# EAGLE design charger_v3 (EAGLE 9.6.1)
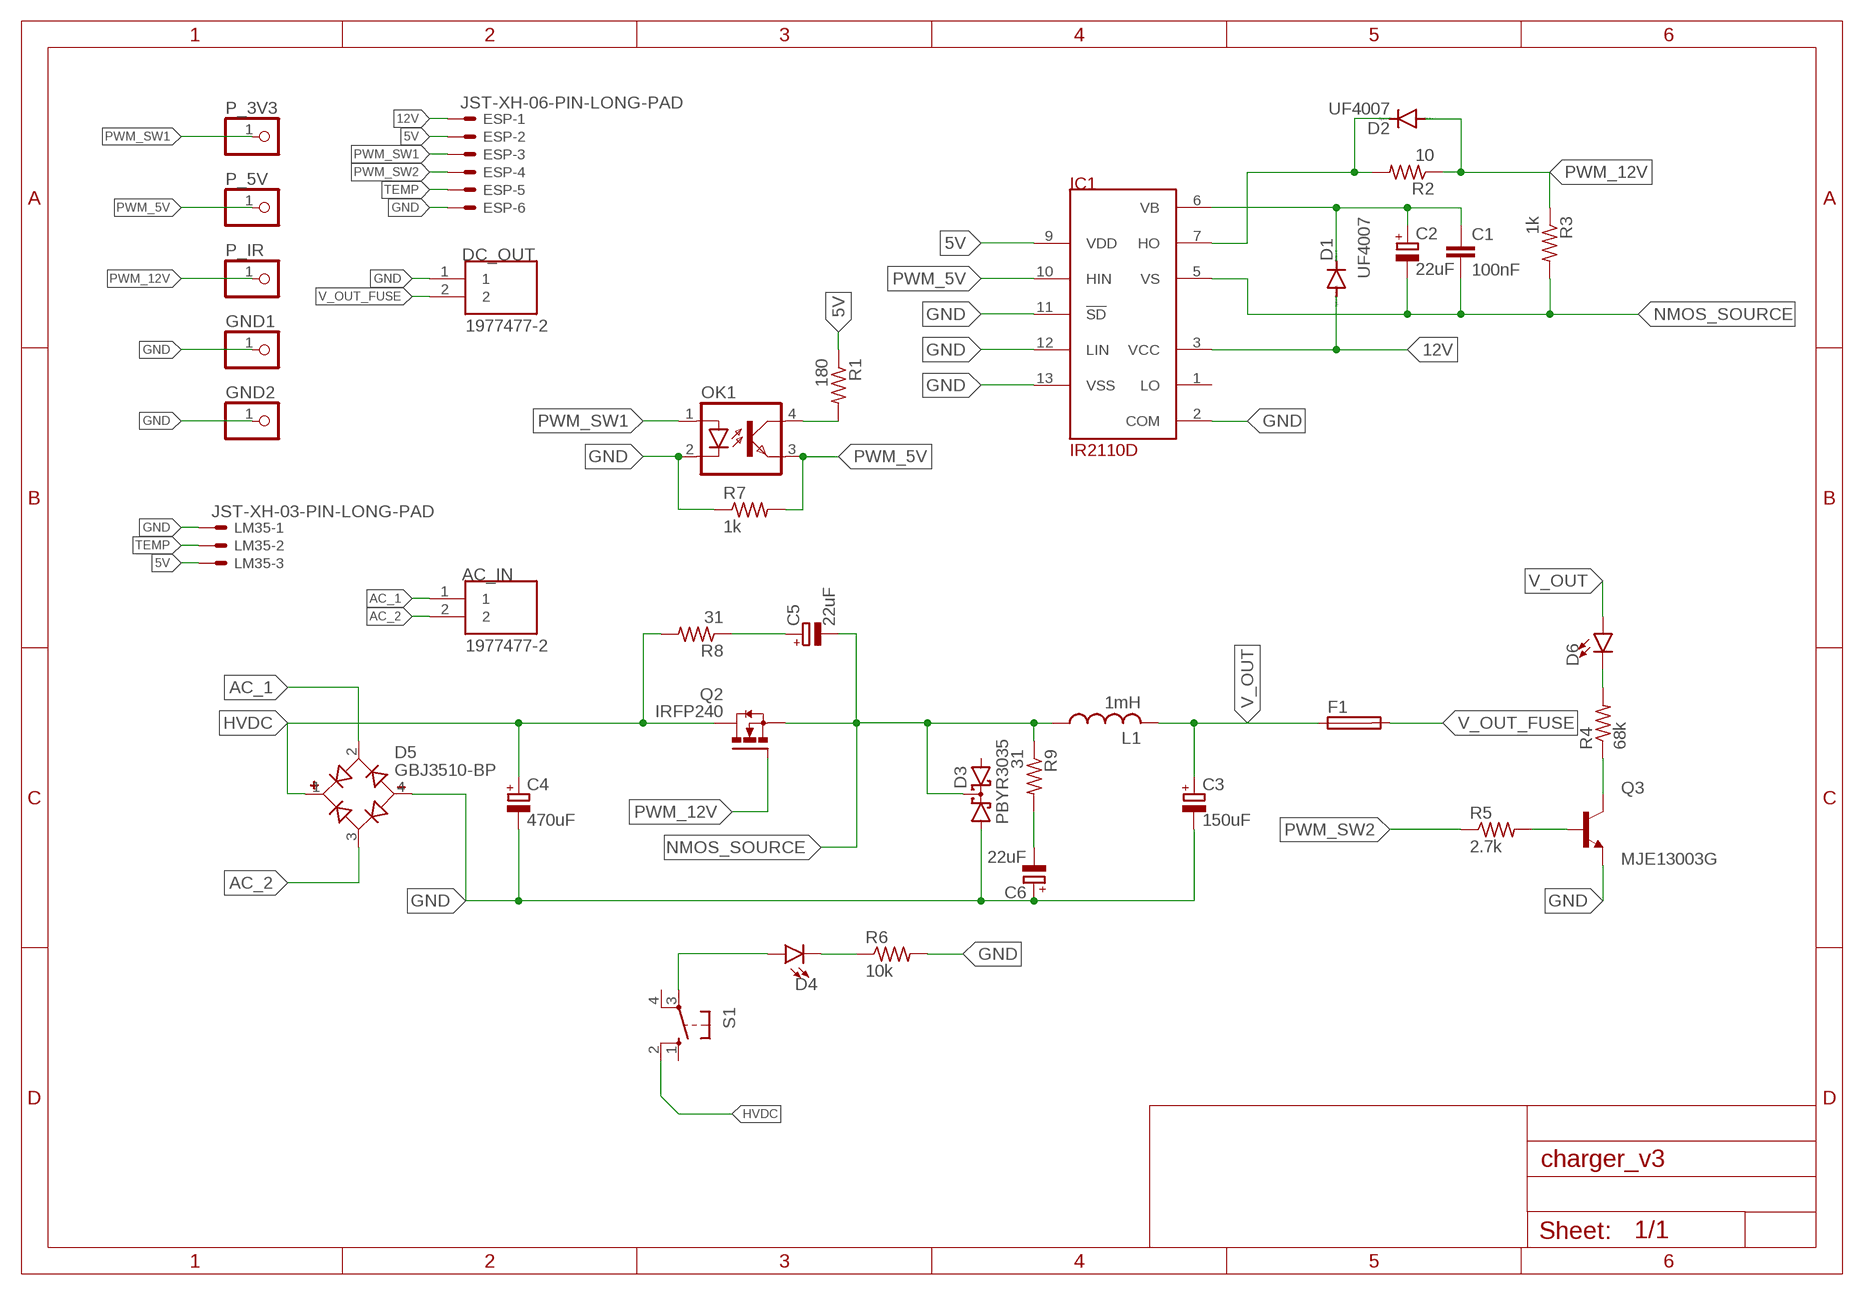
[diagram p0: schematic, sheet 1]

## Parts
AC_IN  1977477-2  [TE_1977477-2]
C1  100nF  C-EU025-025X050  [C025-025X050]
C2  22uF  CPOL-EUE2,5-6E  [E2,5-6E]
C3  150uF  CPOL-EUE7.5-18  [E7,5-18]
C4  470uF  CPOL-EUE10-35  [EB35D]
C5  22uF  CPOL-EUE7.5-18  [E7,5-18]
C6  22uF  CPOL-EUE7.5-18  [E7,5-18]
D1  UF4007  BAS15  [DO34-7]
D2  UF4007  BAS15  [DO34-7]
D3  PBYR3035  [SOT93S]
D4  LED5MM  [LED_5MM]
D5  GBJ3510-BP  [DIOB_GBJ3510-BP]
D6  LED5MM  [LED_5MM]
DC_OUT  1977477-2  [TE_1977477-2]
ESP  JST-XH-06-PIN-LONG-PAD  [JST-XH-06-PACKAGE-LONG-PAD]
F1  FUSEHOLDER  [FUSEHOLDER]
GND1  PINHD-1X1  [1X01]
GND2  PINHD-1X1  [1X01]
IC1  IR2110D  [DIL14]
L1  1mH  L-USTJ7-U1  [TJ7-U1]
LM35  JST-XH-03-PIN-LONG-PAD  [JST-XH-03-PACKAGE-LONG-PAD]
OK1  SFH618A-5  [DIP4]
P_3V3  PINHD-1X1  [1X01]
P_5V  PINHD-1X1  [1X01]
P_IR  PINHD-1X1  [1X01]
Q2  IRFP240  [TO247AC]
Q3  MJE13003G  [TO229P780X300X1364-3]
R1  180  R-US_0204/7  [0204/7]
R2  10  R-US_0204/7  [0204/7]
R3  1k  R-US_0204/7  [0204/7]
R4  68k  R-US_0309/12  [0309/12]
R5  2.7k  R-US_0204/7  [0204/7]
R6  10k  R-US_0204/7  [0204/7]
R7  1k  R-US_0204/7  [0204/7]
R8  31  R-US_0411/15  [0411/15]
R9  31  R-US_0411/15  [0411/15]
S1  10-XX  [B3F-10XX]

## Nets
5V: ESP.2 IC1.9(VDD) LM35.3 R1.1
12V: D1.A ESP.1 IC1.3(VCC)
AC_1 [power]: AC_IN.1 D5.2(AC1)
AC_2 [power]: AC_IN.2 D5.3(AC2)
GND: C3.- C4.- C6.+ D3.A1 D5.4(-) DC_OUT.1 ESP.6 GND1.1 GND2.1 IC1.2(COM) IC1.11(!SD) IC1.12(LIN) IC1.13(VSS) LM35.1 OK1.2(C) Q3.3(E) R6.2 R7.1
HVDC: C4.+ D5.1(+) Q2.2(D) R8.2 S1.2(S1)
N$1: D2.C IC1.7(HO) R2.2
N$2: D4.A S1.3(P)
N$3: Q3.2(C) R4.1
N$4: D6.K(C) R4.2
N$5: Q3.1(B) R5.2
N$6: C5.+ R8.1
N$7: C6.- R9.2
N$8: D4.K(C) R6.1
N$11: OK1.4(COL) R1.2
NMOS_SOURCE: C1.2 C2.- C5.- D3.C IC1.5(VS) L1.1 Q2.3(S) R3.2 R9.1
PWM_5V: IC1.10(HIN) OK1.3(EMIT) P_5V.1 R7.2
PWM_12V [pwm_12]: D2.A P_IR.1 Q2.1(G) R2.1 R3.1
PWM_SW1: ESP.3 OK1.1(A) P_3V3.1
PWM_SW2: ESP.4 R5.1
TEMP: ESP.5 LM35.2
V_OUT: C3.+ D6.A F1.1 L1.2
V_OUT_FUSE [power]: DC_OUT.2 F1.2
VB: C1.1 C2.+ D1.C IC1.6(VB)
Unconnected: D3.A2 IC1.1(LO) S1.1(S) S1.4(P1)

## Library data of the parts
AC_IN DC_OUT = terminal_block_TA:1977477-2: Check availability; AVAILABILITY: In Stock; COMMENT: 1977477-2; DESCRIPTION: Conn Barrier Strip 2 POS 8.25mm Solder ST Thru-Hole 15A/Contact Carton; MF: TE Connectivity; MP: 1977477-2; PACKAGE: None; PRICE: None; PURCHASE-URL: https://pricing.snapeda.com/search/part/1977477-2/?ref=eda
C1 = rcl:C-EU: CAPACITOR, European symbol; SPICEPREFIX: C
C2-C6 = rcl:CPOL-EU: POLARIZED CAPACITOR, European symbol; SPICEPREFIX: C
D1 D2 = diode:BAS15: DIODE
D3 = diode:PBYR3035: Dual DIODE common cathode
D4 D6 = Sparkfun_LED:LED: LED (Generic)
D5 = GBJ3510-BP:GBJ3510-BP: Diode Rectifier Bridge Single 1KV 35A 4-Pin(4+Tab) Case GBJ Bulk/Tube Check availability; AVAILABILITY: In Stock; DESCRIPTION: Bridge Rectifier Single Phase Standard 1 kV Through Hole GBJ; MF: Micro Commercial; MP: GBJ3510-BP; PACKAGE: SIP-4 Micro Commercial Co; PRICE: None; PURCHASE-URL: https://pricing.snapeda.com/search/part/GBJ3510-BP/?ref=eda
ESP = Rembrandt Electronics - JST XH Connectors v1-0:JST-XH-06-PIN: JST XH Connector 2 Pin Wire to board connector. Pitch: 2,54 mm, (0.100") Number of pins: 6 Created by Rembrandt Electronics www.rembrandtelectronics.com
F1 = TA_library:FUSEHOLDER: FUSE HOLDER; MPN: 0031.7701.11; OC_FARNELL: unknown; OC_NEWARK: 04F1224
GND1 GND2 P_3V3 P_5V P_IR = pinhead:PINHD-1X1: PIN HEADER
IC1 = irs:IR2110
L1 = custom_inductor:L-US: INDUCTOR, American symbol; SPICEPREFIX: L
LM35 = Rembrandt Electronics - JST XH Connectors v1-0:JST-XH-03-PIN: JST XH Connector 2 Pin Wire to board connector. Pitch: 2,54 mm, (0.100") Number of pins: 3 Created by Rembrandt Electronics www.rembrandtelectronics.com
OK1 = optocoupler:SFH618?*: Optocoupler, Phototransistor Output, Low Input Current Source: Data sheet; MF: VISHAY/TELEFUNKEN; MPN: SFH618A-5; OC_FARNELL: 1469593; OC_NEWARK: 59K0259
Q2 = IRFP240(TO-247):IRFP240: MOSFET N-CH 200V 20A TO-247AC Check availability; AVAILABILITY: In Stock; DESCRIPTION: N-Channel 200 V 20A (Tc) 150W (Tc) Through Hole TO-247AC; MF: Vishay Siliconix; MP: IRFP240; PACKAGE: TO-247 Vishay Siliconix; PRICE: None
Q3 = MJE13003G:MJE13003G: Bipolar (BJT) Transistor NPN 400V 1.5A 10MHz 1.4W Through Hole TO-225AA Check availability; AVAILABILITY: Not in stock; DESCRIPTION: Bipolar (BJT) Transistor NPN 400 V 1.5 A 10MHz 1.4 W Through Hole TO-126; MF: ON Semiconductor; MP: MJE13003G; PACKAGE: TO-126 ON Semiconductor; PRICE: None
R1-R9 = rcl:R-US_: RESISTOR, American symbol; SPICEPREFIX: R
S1 = switch-omron:10-XX: OMRON SWITCH; MPN: B3F-1000; OC_FARNELL: 176432; OC_NEWARK: 36M3542

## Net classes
0 default: width 0.305 mm
1 power: width 6.985 mm, clearance 0.508 mm to class 0
2 pwm_12: width 0.305 mm, clearance 0.508 mm to class 0, clearance 0.508 mm to class 1

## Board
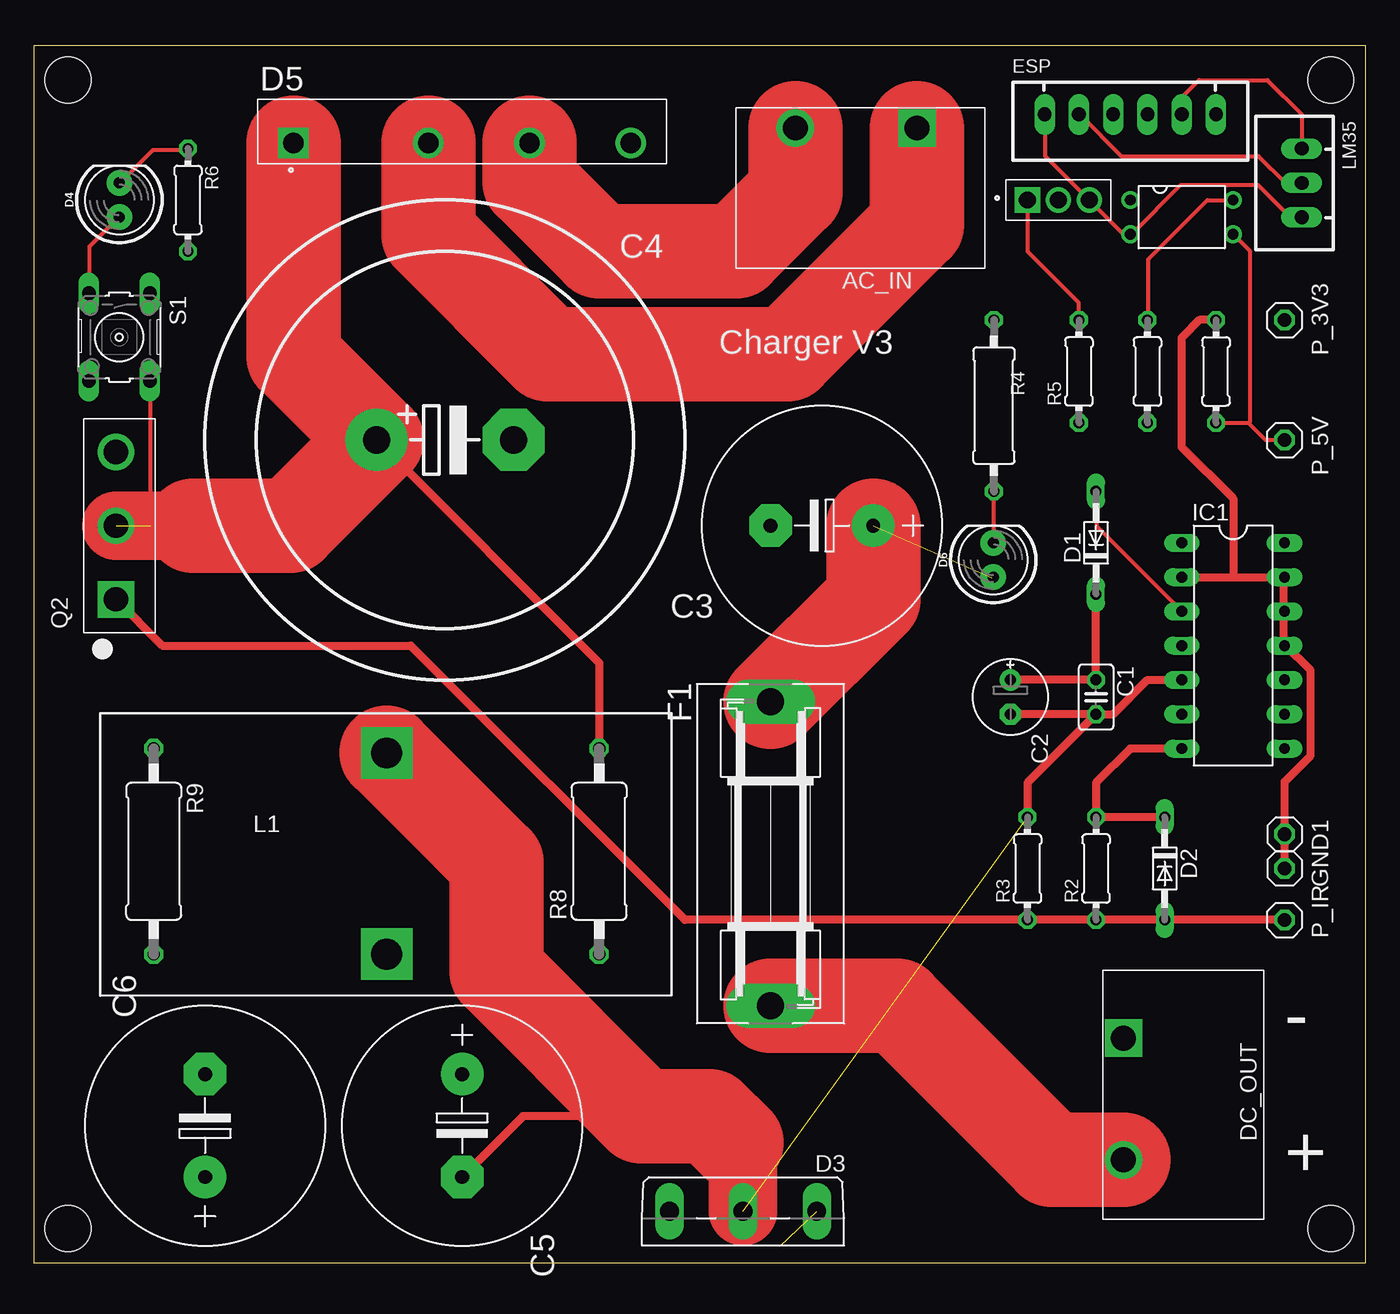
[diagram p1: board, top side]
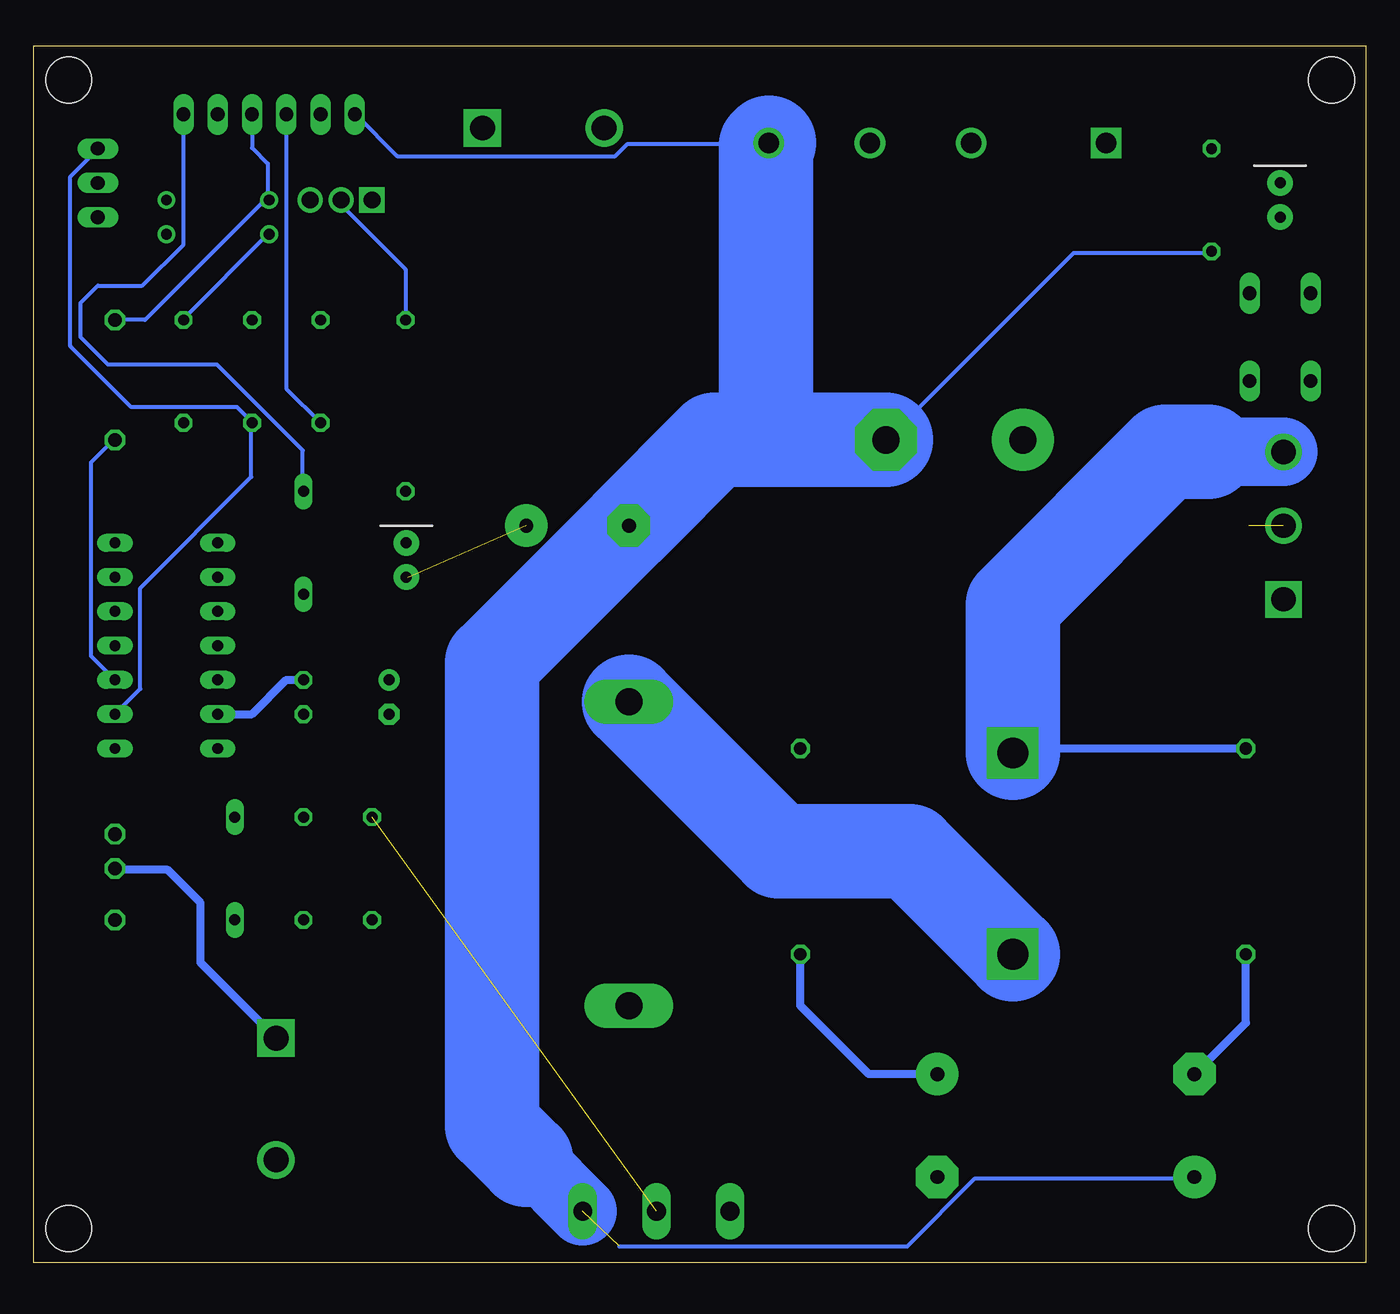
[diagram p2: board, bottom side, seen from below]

Size 98.73 x 90.16 mm. Coordinates in mm from the lower left corner, seen from the top.
Outline: 0,0 98.73,0 98.73,90.16 0,90.16 0,0
Copper layers (1*16): Top 0.035mm / dielectric 1.5mm / Bottom 0.035mm
Design rules "default *": minimum track width 12mil, minimum drill 0.35mm, track to track 12mil, track to pad 12mil, pad to pad 12mil, via to via 12mil, smd to smd 12mil, copper to edge 40mil, drill to drill 6mil, minimum pad ring 10mil, minimum via ring 8mil, stop-mask expansion 4mil, vias tented up to drill 0mil, thermal gap 10mil
Holes 3.4 mm at 2.54,87.63 96.14,87.63 2.54,2.54 96.14,2.54

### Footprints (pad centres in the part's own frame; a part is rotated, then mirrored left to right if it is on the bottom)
TE_1977477-2 = drill 1.85 square: 1 -3.241,-5.334 | drill 1.85: 2 5.781,-5.334
C025-025X050 = drill 0.813 octagon: 1 -1.27,0; 2 1.27,0
E2,5-6E = drill 0.813 pad 1.575: + -1.27,0 | drill 0.813 pad 1.575 octagon: - 1.27,0
E7,5-18 = drill 1.016 pad 3.15: + -3.81,0 | drill 1.016 pad 3.15 octagon: - 3.81,0
EB35D = drill 2.007 pad 4.597: + -5.08,0 | drill 2.007 pad 4.597 octagon: - 5.08,0
DO34-7 = drill 0.813 long: A 3.81,0; C -3.81,0
SOT93S = drill 1.397 long: A1 -5.461,-2.54; A2 5.461,-2.54; C 0,-2.54
LED_5MM = drill 0.813 pad 1.88: A -1.27,0; K 1.27,0
DIOB_GBJ3510-BP = drill 1.51 pad 2.27 square: 1 -12.5,-0.85 | drill 1.51 pad 2.27: 2 -2.5,-0.85; 3 5,-0.85; 4 12.5,-0.85
JST-XH-06-PACKAGE-LONG-PAD = drill 1.016 long: 1 -6.35,0; 2 -3.81,0; 3 -1.27,0; 4 1.27,0; 5 3.81,0; 6 6.35,0
FUSEHOLDER = drill 2.007 pad 3.302 long: 1 -11.252,0; 2 11.252,0
1X01 = drill 1.016 octagon: 1 0,0
DIL14 = drill 0.813 long: 1 -7.62,-3.81; 2 -5.08,-3.81; 3 -2.54,-3.81; 4 0,-3.81; 5 2.54,-3.81; 6 5.08,-3.81; 7 7.62,-3.81; 8 7.62,3.81; 9 5.08,3.81; 10 2.54,3.81; 11 0,3.81; 12 -2.54,3.81; 13 -5.08,3.81; 14 -7.62,3.81
TJ7-U1 = drill 2.286 pad 3.81 square: 1 -6.503,4.826; 2 8.408,4.826
JST-XH-03-PACKAGE-LONG-PAD = drill 1.016 long: 1 -2.54,0; 2 0,0; 3 2.54,0
DIP4 = drill 0.8: 1 -1.27,-3.81; 2 1.27,-3.81; 3 1.27,3.81; 4 -1.27,3.81
TO247AC = drill 1.79 pad 2.69 square: 1 -5.46,0.255 | drill 1.79 pad 2.69: 2 0,0.255; 3 5.46,0.255
TO229P780X300X1364-3 = drill 1.25 square: 1 0,0 | drill 1.25: 2 2.29,0; 3 4.58,0
0204/7 = drill 0.813 octagon: 1 -3.81,0; 2 3.81,0
0309/12 = drill 0.813 octagon: 1 -6.35,0; 2 6.35,0
0411/15 = drill 0.914 octagon: 1 -7.62,0; 2 7.62,0
B3F-10XX = drill 1.016 long: 1 -3.251,2.261; 2 3.251,2.261; 3 -3.251,-2.261; 4 3.251,-2.261

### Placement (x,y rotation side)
AC_IN  62.23,78.74 180 top
C1  78.74,41.91 270 top
C2  72.39,41.91 270 top
C3  58.42,54.61 180 top
C4  30.48,60.96 0 top
C5  31.75,10.16 270 top
C6  12.7,10.16 90 top
D1  78.74,53.34 90 top
D2  83.82,29.21 270 top
D3  52.58,1.27 180 top
D4  6.35,78.74 90 top
D5  31.75,83.82 0 top
D6  71.12,52.07 90 top
DC_OUT  86.11,13.4 270 top
ESP  81.28,85.09 180 top
F1  54.61,30.3 270 top
GND1  92.71,31.75 0 top
GND2  92.71,29.21 0 top
IC1  88.9,45.72 270 top
L1  21.34,31.27 270 top
LM35  93.98,80.01 90 top
OK1  85.09,77.47 270 top
P_3V3  92.71,69.85 90 top
P_5V  92.71,60.96 90 top
P_IR  92.71,25.4 90 top
Q2  6.35,54.61 90 top
Q3  73.66,78.74 0 top
R1  82.55,66.04 90 top
R2  78.74,29.21 90 top
R3  73.66,29.21 90 top
R4  71.17,63.5 270 top
R5  77.47,66.04 90 top
R6  11.43,78.74 270 top
R7  87.63,66.04 270 top
R8  41.91,30.48 90 top
R9  8.89,30.48 270 top
S1  6.35,68.58 270 top

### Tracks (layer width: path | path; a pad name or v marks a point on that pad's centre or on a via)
5V
  Top 0.305: LM35.3 93.98,85.09 91.44,87.63 86.36,87.63 85.09,86.36 ESP.2
  Bottom 0.305: IC1.9 90.83,42.52 90.83,49.99 82.6,58.22 82.6,62.18 R1.1 82.6,62.33 83.67,63.4 91.49,63.4 96.01,67.92 96.01,80.47 94.03,82.45 LM35.3
12V
  Top 0.305: IC1.3 78.79,54.56 78.79,57.15 D1.A
  Bottom 0.305: ESP.1 87.63,75.44 90.68,72.39 93.98,72.39 95.25,71.12 95.25,68.58 93.22,66.55 85.14,66.55 78.79,60.2 78.79,57.15 D1.A
AC_1
  Top 6.985: AC_IN.1 65.47,76.9 55.88,67.31 38.1,67.31 29.25,76.16 D5.2
AC_2
  Top 6.985: AC_IN.2 56.45,79.31 52.07,74.93 41.91,74.93 36.75,80.09 D5.3
GND  (1 unrouted)
  Top 0.305: 54.56,54.71 C3.- | 35.66,60.96 C4.- | GND2.1 92.81,29.26 92.81,31.7 GND1.1 92.81,31.85 92.81,35.81 94.49,37.49 94.49,44.04 92.81,45.72 IC1.11 92.66,45.72 92.66,48.16 IC1.12 92.66,48.31 92.66,50.75 IC1.13 92.66,50.9 | ESP.6 74.98,85.04 74.98,81.99 78.18,78.79 Q3.3 78.33,78.64 80.77,76.2 OK1.2 81.38,76.2 85.04,79.86 90.73,79.86 93.02,77.57 93.88,77.57 LM35.1
  Top 0.61: GND2.1 92.71,35.64 94.64,37.57 94.64,43.89 92.81,45.72 | IC1.11 92.66,45.77 92.66,50.9 92.56,50.8 88.9,50.8 | 88.9,50.8 88.9,56.62 85.09,60.43 85.09,68.53 86.41,69.85 R7.1 | IC1.2 88.9,50.8
  Bottom 0.305: R6.2 11.43,74.83 21.64,74.83 35.51,60.96 C4.- | 44.2,82.91 D5.4 44.35,82.91 54.71,82.91 55.63,81.99 71.78,81.99 74.83,85.04 ESP.6 | R7.1 87.63,69.95 81.38,76.2 OK1.2 | 55.32,1.22 33.98,1.22 28.96,6.25 12.8,6.25 C6.+
  Bottom 0.61: GND2.1 92.61,29.11 88.8,29.11 86.36,26.67 86.36,22.23 DC_OUT.1
  Bottom 3.81: 64.39,10.16 64.77,10.16
  Bottom 5.08: D3.A1 61.85,7.62 62.23,7.62
  Bottom 6.985: 62.23,7.62 64.77,10.16 64.77,44.45 C3.- 48.26,60.96 44.45,60.96 | C4.- 44.45,60.96 | D5.4 44.45,82.77 44.45,60.96
HVDC  (1 unrouted)
  Top 0.305: 8.69,54.61 8.69,65.23 S1.2
  Top 0.61: R8.2 41.91,44.45 C4.+
  Top 5.08: Q2.2 11.81,54.61
  Top 6.985: D5.1 19.25,67.11 C4.+ 19.05,54.61 11.81,54.61
N$1
  Top 0.61: IC1.7 81.28,38.1 78.74,35.56 R2.2 D2.C
N$2
  Top 0.305: S1.3 4.12,71.93 4.12,75.29 6.25,77.42 D4.A
N$3
  Bottom 0.305: R4.1 71.17,73.61 75.89,78.33 75.89,78.64 Q3.2
N$4
  Top 0.305: R4.2 71.17,53.34 D6.K
N$5
  Top 0.305: Q3.1 73.66,74.93 77.42,71.17 77.42,69.95 R5.2
N$6
  Bottom 0.61: C5.+ 36.83,13.97 41.91,19.05 R8.1
N$7
  Bottom 0.61: C6.- 8.89,17.78 R9.2
N$8
  Top 0.305: R6.1 11.43,82.45 8.84,82.45 6.4,80.01 D4.K
N$11
  Top 0.305: OK1.4 87,78.74 82.6,74.35 82.6,72.75 82.6,72.39 82.6,69.95 R1.2
NMOS_SOURCE  (1 unrouted)
  Top 0.61: C1.2 80.01,40.64 82.55,43.18 IC1.5 | C1.2 C2.- | C1.2 73.66,35.56 R3.2 | 45.02,10.86 36.26,10.86 C5.-
  Top 5.08: D3.C 52.58,8.38 52.07,8.89
  Top 6.985: L1.1 34.29,29.64 34.29,21.59 45.02,10.86 50.1,10.86 52.07,8.89
  Bottom 0.61: R9.1 25.83,38.1 L1.1
  Bottom 5.08: Q2.3 11.68,60.07
  Bottom 6.985: L1.1 26.16,48.77 14.86,60.07 11.68,60.07
PWM_5V
  Top 0.305: OK1.3 90.12,74.98 90.12,62.28 90.04,62.2 | 90.04,62.2 90.02,62.23 R7.2 | P_5V.1 91.29,60.96 90.04,62.2
  Bottom 0.305: IC1.10 94.49,44.96 94.49,59.28 92.81,60.96 P_5V.1
PWM_12V
  Top 0.305: R2.1 D2.A
  Top 0.61: P_IR.1 D2.A R3.1 48.26,25.4 27.94,45.72 9.53,45.72 Q2.1
PWM_SW1
  Bottom 0.305: ESP.3 82.55,82.6 81.38,81.43 81.38,78.79 OK1.1 81.53,78.79 90.47,69.85 P_3V3.1
PWM_SW2
  Bottom 0.305: ESP.4 80.01,64.77 R5.1
TEMP
  Top 0.305: LM35.2 92.76,80.01 90.78,81.99 80.62,81.99 77.57,85.04 ESP.5
V_OUT  (1 unrouted)
  Top 6.985: F1.1 62.23,49.17 C3.+
  Bottom 0.305: 71.02,50.75 D6.A
  Bottom 6.985: L1.2 33.78,30.48 43.54,30.48 F1.1
V_OUT_FUSE
  Top 6.985: F1.2 64.01,19.05 75.44,7.62 DC_OUT.2
VB
  Top 0.61: D1.C C1.1 C2.+
  Bottom 0.61: IC1.6 82.55,40.64 80.01,43.18 C1.1

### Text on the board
tPlace: - | +
tNames: Charger V3

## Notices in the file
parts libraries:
Sparkfun_LED: Licensing: Creative Commons ShareAlike 4.0 International - https://creativecommons.org/licenses/by-sa/4.0
